[IBIS VER]   4.1
[File Name]   f29h85xpzs.ibs
[File Rev]   1.0
[Date]   May 06, 2024
[Source]   File originated at Texas Instruments
[Copyright]   (c) 2012, Texas Instruments Inc.
[Component]   f29h85xpzs
[Manufacturer]  Texas Instruments
[Package]
| Variable   Typ   Min   Max
R_pkg   2.16E-01   8.19E-02   3.21E-01
L_pkg   3.14E-09   1.61E-09   4.25E-09
C_pkg   1.08E-13   5.34E-14   3.30E-13
[Pin]   signal_name   model_name   R_pin   L_pin   C_pin
1   GPIO15   BQ33100HYPBFZ_PMB_5FS_LC_7LM   2.36E-01   3.63E-09   3.17E-13
2   GPIO16   BCF33100DSHYPBFZ_USF_7LM   2.32E-01   3.55E-09   1.55E-13
3   VDDIO   NC   2.22E-01   3.44E-09   1.06E-13
4   GPIO17   BCF33100DSHYPBFZ_USF_7LM   2.19E-01   3.37E-09   1.03E-13
5   VDD   NC   1.26E-01   2.56E-09   1.03E-13
6   VDD   NC   1.44E-01   2.67E-09   1.01E-13
7   VDDIO   NC   2.99E-01   3.91E-09   9.60E-14
8   GPIO18   BQ33100HYPBFZ_PMB_5FS_LC_7LM   2.79E-01   3.70E-09   9.32E-14
9   GPIO22   BQ33100HYPBFZ_PMB_5FS_LC_7LM   2.67E-01   3.56E-09   9.05E-14
10   B9,GPIO233   BCF33100DSHYPBFZ_USF_7LM   2.79E-01   3.62E-09   8.80E-14
11   B8,GPIO232   BCF33100DSHYPBFZ_USF_7LM   2.61E-01   3.43E-09   8.53E-14
12   A7/E25,GPIO225   BCF33100DSHYPBFZ_USF_7LM   2.73E-01   3.50E-09   8.28E-14
13   A6/E24,GPIO224   BCF33100DSHYPBFZ_USF_7LM   2.58E-01   3.33E-09   8.01E-14
14   VDDA   NC   1.50E-01   2.48E-09   8.54E-14
15   VSSA   NC   1.42E-01   2.46E-09   8.78E-14
16   B3/D27   ICF33SHYPB_LC_7LM   2.76E-01   3.60E-09   8.80E-14
17   B2/D26   ICF33SHYPB_LC_7LM   2.57E-01   3.48E-09   9.04E-14
18   VREFLOAB   NC   1.30E-01   2.47E-09   9.51E-14
19   VREFHIAB   NC   8.60E-02   2.15E-09   9.95E-14
20   A15/B15/C15/D15/E15   ICF33SHYPB_LC_7LM   2.27E-01   3.35E-09   9.80E-14
21   A14/B14/C14/D14/E14   ICF33SHYPB_LC_7LM   2.18E-01   3.32E-09   1.00E-13
22   B1/C27   ICF33SHYPB_LC_7LM   2.14E-01   3.33E-09   1.03E-13
23   B0/C26/VDAC   ICF33SHYPB_LC_7LM   2.16E-01   3.38E-09   1.06E-13
24   A1/C25   ICF33SHYPB_LC_7LM   2.24E-01   3.49E-09   1.55E-13
25   A0/C24/DACA_OUT   ICF33SHYPB_LC_7LM   2.38E-01   3.65E-09   3.17E-13
26   C0/E28   ICF33SHYPB_LC_7LM   2.38E-01   3.71E-09   3.30E-13
27   C1/E29   ICF33SHYPB_LC_7LM   2.23E-01   3.55E-09   1.61E-13
28   D0/B24   ICF33SHYPB_LC_7LM   2.13E-01   3.43E-09   1.57E-13
29   D1/B25   ICF33SHYPB_LC_7LM   2.11E-01   3.37E-09   1.07E-13
30   E0/A24/DACC_OUT   ICF33SHYPB_LC_7LM   2.15E-01   3.36E-09   1.05E-13
31   E1/A25   ICF33SHYPB_LC_7LM   2.23E-01   3.39E-09   1.02E-13
32   VREFLOCDE   NC   1.20E-01   2.50E-09   1.01E-13
33   VREFHICDE   NC   8.67E-02   2.18E-09   1.01E-13
34   D2/B26   ICF33SHYPB_LC_7LM   2.45E-01   3.44E-09   9.40E-14
35   D3/B27   ICF33SHYPB_LC_7LM   2.63E-01   3.55E-09   9.15E-14
36   VSSA   NC   1.41E-01   2.50E-09   9.12E-14
37   VDDA   NC   1.48E-01   2.51E-09   8.87E-14
38   E4/A28,GPIO246   BCF33100DSHYPBFZ_USF_7LM   2.15E-01   3.02E-09   8.30E-14
39   E5/A29,GPIO247   BCF33100DSHYPBFZ_USF_7LM   2.13E-01   2.97E-09   8.02E-14
40   C8,GPIO238   BCF33100DSHYPBFZ_USF_7LM   2.15E-01   2.94E-09   7.76E-14
41   C9,GPIO239   BCF33100DSHYPBFZ_USF_7LM   2.21E-01   2.95E-09   7.49E-14
42   GPIO222/TDI   BCF33100DSHYPBFZ_USF_7LM   2.14E-01   2.85E-09   7.21E-14
43   GPIO223/TDO   BCPF335585DSHYPBFZ_USF_7LM   2.21E-01   2.87E-09   6.95E-14
44   VDDIO   NC   2.31E-01   2.91E-09   6.69E-14
45   VDD   NC   8.84E-02   1.69E-09   6.87E-14
46   VDD3VFL   NC   8.72E-02   1.64E-09   6.59E-14
47   TMS   BCF3355DSHYPBFZ_TMS_USF_7LM   2.47E-01   2.91E-09   5.89E-14
48   TCK   IQ0442FS_40P60P_3X2_USF_7LM   2.66E-01   3.03E-09   5.64E-14
49   VDD   NC   9.94E-02   1.61E-09   5.88E-14
50   GPIO41   BCF33100DSHYPBFZ_CORNER_USF_7LM   2.35E-01   2.69E-09   1.01E-13
51   GPIO219/ERRORSTS   BCF33100DSHYPBFZ_CORNER_USF_7LM   2.61E-01   3.84E-09   3.17E-13
52   VDD3VFL   NC   1.16E-01   2.61E-09   1.61E-13
53   GPIO58   BCF33100DSHYPBFZ_USF_7LM   3.21E-01   4.25E-09   1.07E-13
54   GPIO59   BCF3385DSHYPBFZ_USF_7LM   2.98E-01   4.02E-09   1.04E-13
55   VDD   NC   1.04E-01   2.39E-09   1.06E-13
56   GPIO60   BCF33100DSHYPBFZ_USF_7LM   2.72E-01   3.72E-09   9.83E-14
57   GPIO61   BCF33100DSHYPBFZ_USF_7LM   2.85E-01   3.79E-09   9.59E-14
58   GPIO62   BCF33100DSHYPBFZ_USF_7LM   2.67E-01   3.60E-09   9.31E-14
59   GPIO63   BCF33100DSHYPBFZ_USF_7LM   2.50E-01   3.43E-09   9.04E-14
60   GPIO64   BCF3385DSHYPBFZ_USF_7LM   2.37E-01   3.28E-09   8.77E-14
61   GPIO65   BCF33100DSHYPBFZ_USF_7LM   2.26E-01   3.15E-09   8.50E-14
62   GPIO66   BCF33100DSHYPBFZ_USF_7LM   2.22E-01   3.07E-09   8.24E-14
63   VDDIO   NC   2.20E-01   3.01E-09   7.97E-14
64   GPIO127   BCF33100DSHYPBFZ_USF_7LM   2.25E-01   3.10E-09   8.24E-14
65   VREGENZ   IQ0440FS_VREGENZ_PU_7LM   2.22E-01   3.11E-09   8.49E-14
66   VDD   NC   8.19E-02   2.00E-09   9.14E-14
67   VDDOSC   NC   2.19E-01   3.17E-09   9.01E-14
68   GPIO221,X2   BCPF335585DSHYPBFZ_USF_7LM   2.18E-01   3.20E-09   9.27E-14
69   VSSOSC   NC   2.18E-01   3.24E-09   9.53E-14
70   GPIO220,X1   BCPF335585DSHYPBFZ_USF_7LM   2.22E-01   3.31E-09   9.79E-14
71   XRSn   BQ0491FS_3X2_USF_7LM   2.21E-01   3.34E-09   1.00E-13
72   GPIO38   BCF33100DSHYPBFZ_USF_7LM   2.27E-01   3.44E-09   1.03E-13
73   VDDIO   NC   2.31E-01   3.51E-09   1.06E-13
74   GPIO42   BCPF335585DSHYPBFZ_USF_7LM   2.32E-01   3.56E-09   1.55E-13
75   GPIO43   BCF33100DSHYPBFZ_CORNER_USF_7LM   2.45E-01   3.71E-09   3.17E-13
76   GPIO70   BCF3385DSHYPBFZ_CORNER_7LM   2.49E-01   3.81E-09   3.30E-13
77   GPIO71   BCF33100DSHYPBFZ_USF_7LM   2.34E-01   3.64E-09   1.61E-13
78   VDD   NC   1.22E-01   2.68E-09   1.59E-13
79   VDDIO   NC   2.26E-01   3.49E-09   1.07E-13
80   GPIO72   BCF33100DSHYPBFZ_USF_7LM   2.19E-01   3.39E-09   1.05E-13
81   GPIO84   BCF33100DSHYPBFZ_USF_7LM   2.56E-01   3.66E-09   1.02E-13
82   GPIO31   BCF33100DSHYPBFZ_USF_7LM   2.54E-01   3.60E-09   9.95E-14
83   GPIO30   BCF3355DSHYPBFZ_USF_7LM   2.49E-01   3.51E-09   9.68E-14
84   GPIO29   BQ33100HYPBFZ_PMB_5FS_LC_7LM   2.43E-01   3.43E-09   9.40E-14
85   GPIO26   BCF33100DSHYPBFZ_USF_7LM   2.72E-01   3.62E-09   9.16E-14
86   GPIO25   BCF33100DSHYPBFZ_USF_7LM   2.54E-01   3.43E-09   8.87E-14
87   GPIO23   BQ33100HYPBFZ_PMB_5FS_LC_7LM   2.45E-01   3.31E-09   8.59E-14
88   GPIO0   BCF33100DSHYPBFZ_USF_7LM   2.47E-01   3.29E-09   8.32E-14
89   GPIO1   BCF33100DSHYPBFZ_USF_7LM   2.34E-01   3.14E-09   8.04E-14
90   GPIO2   BCF33100DSHYPBFZ_USF_7LM   2.23E-01   3.01E-09   7.76E-14
91   GPIO3   BCF33100DSHYPBFZ_USF_7LM   2.16E-01   2.91E-09   7.49E-14
92   GPIO4   BCF33100DSHYPBFZ_USF_7LM   2.13E-01   2.84E-09   7.21E-14
93   GPIO5   BCF33100DSHYPBFZ_USF_7LM   2.12E-01   2.79E-09   6.94E-14
94   GPIO6   BCF3355DSHYPBFZ_USF_7LM   2.16E-01   2.78E-09   6.68E-14
95   VDD   NC   1.19E-01   1.94E-09   6.61E-14
96   GPIO8   BCF33100DSHYPBFZ_USF_7LM   2.15E-01   2.69E-09   6.13E-14
97   GPIO9   BCF3385DSHYPBFZ_USF_7LM   2.22E-01   2.71E-09   5.87E-14
98   GPIO10   BQ33100HYPBFZ_PMB_5FS_LC_7LM   2.26E-01   2.70E-09   5.60E-14
99   GPIO11   BCF33100DSHYPBFZ_USF_7LM   2.36E-01   2.74E-09   5.34E-14
100   GPIO12   BCF33100DSHYPBFZ_CORNER_USF_7LM   2.47E-01   2.79E-09   1.02E-13
| End of package information
|   Component BCF33100DSHYPBFZ_7LM
[Component]   BCF33100DSHYPBFZ_7LM
[Manufacturer]  IO Methodology Inc.
[Package]
|   typ   min   max
R_pkg   0   0   0
L_pkg   0   0   0
C_pkg   0   0   0
[Pin]   signal_name  model_name   R_pin   L_pin   C_pin
VSS   VSS   GND
VDDS   VDDS   POWER
PAD   PAD   BCF33100DSHYPBFZ_7LM
[Model Selector] BCF33100DSHYPBFZ_7LM
WK_PU_ON_3P3  Cell operated at 3.3(nom)
|WK_PU_ON_3P3; WEAK_PULLUP_ON
WK_PD_ON_3P3  Cell operated at 3.3(nom)
|WK_PD_ON_3P3; WEAK_PULLDOWN_ON
DRIVER_MODE_3P3  Cell operated at 3.3(nom)
|DRIVER_MODE_3P3
RECEIVER_MODE_3P3  Cell operated at 3.3(nom)
|   Component BCF33100DSHYPBFZ_USF_7LM
[Component]   BCF33100DSHYPBFZ_USF_7LM
[Manufacturer]  Texas Instruments
[Package]
| variable   typ   min   max
R_pkg   0.0   0.0   0.0
L_pkg   0.0H   0.0H   0.0H
C_pkg   0.0F   0.0F   0.0F
[Pin]  signal_name   model_name   R_pin   L_pin   C_pin
PAD   PAD   BCF33100_USF_7LM_IO_3.3V   0   0   0
VDDS   VDDS   Power   0   0   0
VSS   VSS   Gnd   0   0   0
[Model Selector] BCF33100DSHYPBFZ_USF_7LM
BCF33100_USF_7LM_IO_3.3V I/O model with 3.3V supply
|   Component BCF33100DSHYPBFZ_CORNER_USF_7LM
[Component]   BCF33100DSHYPBFZ_CORNER_USF_7LM
[Manufacturer]  Texas Instruments
[Package]
| variable   typ   min   max
R_pkg   0.0   0.0   0.0
L_pkg   0.0H   0.0H   0.0H
C_pkg   0.0F   0.0F   0.0F
[Pin]  signal_name   model_name   R_pin   L_pin   C_pin
PAD   PAD   BCF33100_CORNER_7LM_IO_3.3V   0   0   0
VDDS   VDDS   Power   0   0   0
VSS   VSS   Gnd   0   0   0
[Model Selector] BCF33100DSHYPBFZ_CORNER_USF_7LM
BCF33100_CORNER_7LM_IO_3.3V  I/O model with 3.3V supply
|   Component BCF3355DSHYPBFZ_TMS_USF_7LM
[Component]   BCF3355DSHYPBFZ_TMS_USF_7LM
[Manufacturer]  Texas Instruments
[Package]
| variable   typ   min   max
R_pkg   0.0   0.0   0.0
L_pkg   0.0H   0.0H   0.0H
C_pkg   0.0F   0.0F   0.0F
[Pin]  signal_name   model_name   R_pin   L_pin   C_pin
PAD   PAD   BCF3355_TMS_7LM_IO_3.3V   0   0   0
VDDS   VDDS   Power   0   0   0
VSS   VSS   Gnd   0   0   0
[Model Selector] BCF3355DSHYPBFZ_TMS_USF_7LM
BCF3355_TMS_7LM_IO_3.3V I/O model with 3.3V supply
|   Component IQ0442FS_40P60P_3X2_USF_7LM
[Component]   IQ0442FS_40P60P_3X2_USF_7LM
[Manufacturer]  Texas Instruments
[Package]
| variable   typ   min   max
R_pkg   0.0   0.0   0.0
L_pkg   0.0H   0.0H   0.0H
C_pkg   0.0F   0.0F   0.0F
[Pin]  signal_name   model_name   R_pin   L_pin   C_pin
PAD   PAD   IQRX_3.3V   0   0   0
VDDS   VDDS   Power   0   0   0
VSS   VSS   Gnd   0   0   0
[Model Selector] IQ0442FS_40P60P_3X2_USF_7LM
IQRX_3.3V I/O model with 3.3V supply
|   Component BCF3355DSHYPBFZ_USF_7LM
[Component]   BCF3355DSHYPBFZ_USF_7LM
[Manufacturer]  Texas Instruments
[Package]
| variable   typ   min   max
R_pkg   0.0   0.0   0.0
L_pkg   0.0H   0.0H   0.0H
C_pkg   0.0F   0.0F   0.0F
[Pin]  signal_name   model_name   R_pin   L_pin   C_pin
PAD   PAD   BCF3355_USF_7LM_IO_3.3V   0   0   0
VDDS   VDDS   Power   0   0   0
VSS   VSS   Gnd   0   0   0
[Model Selector] BCF3355DSHYPBFZ_USF_7LM
BCF3355_USF_7LM_IO_3.3V I/O model with 3.3V supply
|   Component BCF3385DSHYPBFZ_CORNER_7LM
[Component]   BCF3385DSHYPBFZ_CORNER_7LM
[Manufacturer]  IO Methodology Inc.
[Package]
|   typ   min   max
R_pkg   0   0   0
L_pkg   0   0   0
C_pkg   0   0   0
[Pin]   signal_name  model_name   R_pin   L_pin   C_pin
VSS   VSS   GND
VDDS   VDDS   POWER
PAD   PAD   BCF3385DSHYPBFZ_CORNER_7LM
[Model Selector] BCF3385DSHYPBFZ_CORNER_7LM
WK_PU_ON_3P3_BCF3385DSHYPBFZ_CORNER_7LM  Cell operated at 3.3(nom)
|WK_PU_ON_3P3; WEAK_PULLUP_ON
WK_PD_ON_3P3_BCF3385DSHYPBFZ_CORNER_7LM  Cell operated at 3.3(nom)
|WK_PD_ON_3P3; WEAK_PULLDOWN_ON
DRIVER_MODE_3P3_BCF3385_CORNER_7LM Cell operated at 3.3(nom)
|DRIVER_MODE_3P3
RECEIVER_MODE_3P3_BCF3385_CORNER_7LM  Cell operated at 3.3(nom)
|   Component BCF3385DSHYPBFZ_USF_7LM
[Component]   BCF3385DSHYPBFZ_USF_7LM
[Manufacturer]  Texas Instruments
[Package]
| variable   typ   min   max
R_pkg   0.0   0.0   0.0
L_pkg   0.0H   0.0H   0.0H
C_pkg   0.0F   0.0F   0.0F
[Pin]  signal_name   model_name   R_pin   L_pin   C_pin
PAD   PAD   BCF3385_USF_7LM_IO_3.3V   0   0   0
VDDS   VDDS   Power   0   0   0
VSS   VSS   Gnd   0   0   0
[Model Selector] BCF3385DSHYPBFZ_USF_7LM
BCF3385_USF_7LM_IO_3.3V I/O model with 3.3V supply
|   Component BCPF335585DSHYPBFZ_USF_7LM
[Component]   BCPF335585DSHYPBFZ_USF_7LM
[Manufacturer]  Texas Instruments
[Package]
| variable   typ   min   max
R_pkg   0.0   0.0   0.0
L_pkg   0.0H   0.0H   0.0H
C_pkg   0.0F   0.0F   0.0F
[Pin]  signal_name   model_name   R_pin   L_pin   C_pin
PAD   PAD   BCPF335585DSHYPBFZ_USF_7LM   0   0   0
VDDS   VDDS   Power   0   0   0
VSS   VSS   Gnd   0   0   0
[Model Selector]   BCPF335585DSHYPBFZ_USF_7LM
BCPF335585_7LM_IO_DS0_3.3V   I/O model DS 0 with 3.3V supply
BCPF335585_7LM_IO_DS1_3.3V   I/O model DS 1 with 3.3V supply
|   Component BQ0491FS_3X2_USF_7LM
[Component]   BQ0491FS_3X2_USF_7LM
[Manufacturer]  Texas Instruments
[Package]
| variable   typ   min   max
R_pkg   0.0   0.0   0.0
L_pkg   0.0H   0.0H   0.0H
C_pkg   0.0F   0.0F   0.0F
[Pin]  signal_name   model_name   R_pin   L_pin   C_pin
PAD   PAD   BQ0491FS_3X2_USF_7LM   0   0   0
VDDS   VDDS   Power   0   0   0
VSS   VSS   Gnd   0   0   0
[Model Selector]   BQ0491FS_3X2_USF_7LM
BQ0491_3X2_USF_7LM_IO_15p_3p3   I/O open drain model with C_fixture 15pF for 3.3V supply
BQ0491_3X2_USF_7LM_IO_50p_3p3   I/O open drain model with C_fixture 50pF for 3.3V supply
BQ0491_3X2_USF_7LM_IO_100p_3p3   I/O open drain model with C_fixture 100pF for 3.3V supply
BQ0491_3X2_USF_7LM_IO_150p_3p3   I/O open drain model with C_fixture 150pF for 3.3V supply
|   Component BQ33100HYPBFZ_PMB_5FS_LC_7LM
[Component]   BQ33100HYPBFZ_PMB_5FS_LC
[Manufacturer]  Texas Instruments
[Package]
| variable   typ   min   max
R_pkg   0.0   0.0   0.0
L_pkg   0.0H   0.0H   0.0H
C_pkg   0.0F   0.0F   0.0F
[Pin]  signal_name   model_name   R_pin   L_pin   C_pin
Pin1   PAD   BQ33100HYPBFZ_PMB_5FS_LC_7LM   0   0   0
Pin2   VDDS   Power   0   0   0
Pin3   VSS   Gnd   0   0   0
[Model Selector]   BQ33100HYPBFZ_PMB_5FS_LC_7LM
BQ33_PMB_IO_M0_D0   I/O model with Mode = 0 and Drive = 0
BQ33_PMB_IO_M0_D1   I/O model with Mode = 0 and Drive = 1
BQ33_PMB_IO_M1_D0   I/O model with Mode = 1 and Drive = 0
BQ33_PMB_IO_M1_D1   I/O model with Mode = 1 and Drive = 1
|   Component IQ0440FS_VREGENZ_PU_7LM
[Component]   IQ0440FS_VREGENZ_PU_7LM
[Manufacturer]  Texas Instruments
[Package]
|   typ   min   max
R_pkg   0   0   0
L_pkg   0   0   0
C_pkg   0   0   0
[Pin]   signal_name  model_name   R_pin   L_pin   C_pin
VSS   VSS   GND
VDDS   VDDS   POWER
PAD   PAD   IQ0440FS_VREGENZ_PU_7LM
[Model Selector] IQ0440FS_VREGENZ_PU_7LM
WK_PD_ON_3P3_IQ0440FS_VREGENZ_PU_7LM Cell operated at 3.3(nom)
|WK_PD_ON_3P3; WEAK_PULLDOWN_ON
RECEIVER_MODE_3P3_IQ0440FS_VREGENZ  Cell operated at 3.3(nom)
|   Component ICF33SHYPB_LC_7LM
[Component]   ICF33SHYPB_LC_7LM
[Manufacturer]   Texas Instruments
[Package]
|  variable   typ   min   max
R_pkg   0   0   0
L_pkg   0   0   0
C_pkg   0   0   0
[Pin]   signal_name   model_name   R_pin   L_pin   C_pin
VSS   VSS   GND
VDDS   VDDS   POWER
PAD   PAD   ICF33SHYPB_LC_7LM
[Model Selector] ICF33SHYPB_LC_7LM
RECEIVER_MODE_3P3_ICF_7LM  Cell operated at 3.3(nom)
|RECEIVER_MODE_3P3_ICF_7LM; RECEIVER_MODE
WK_PU_ON_3P3_ICF_7LM  Cell operated at 3.3(nom)
|WK_PU_ON_3P3_ICF_7LM; WEAK_PULLUP_ON
WK_PD_ON_3P3_ICF_7LM  Cell operated at 3.3(nom)
| Models and submodels in the file (29): WK_PU_ON_3P3 (Input), WK_PD_ON_3P3 (Input), DRIVER_MODE_3P3 (I/O), RECEIVER_MODE_3P3 (Input), BCF33100_USF_7LM_IO_3.3V (I/O), BCF33100_CORNER_7LM_IO_3.3V (I/O), BCF3355_TMS_7LM_IO_3.3V (I/O), IQRX_3.3V (Input), BCF3355_USF_7LM_IO_3.3V (I/O), WK_PU_ON_3P3_BCF3385DSHYPBFZ_CORNER_7LM (Input), WK_PD_ON_3P3_BCF3385DSHYPBFZ_CORNER_7LM (Input), DRIVER_MODE_3P3_BCF3385_CORNER_7LM (I/O), RECEIVER_MODE_3P3_BCF3385_CORNER_7LM (Input), BCF3385_USF_7LM_IO_3.3V (I/O), BCPF335585_7LM_IO_DS0_3.3V (I/O), BCPF335585_7LM_IO_DS1_3.3V (I/O), BQ0491_3X2_USF_7LM_IO_15p_3p3 (I/O_open_drain), BQ0491_3X2_USF_7LM_IO_50p_3p3 (I/O_open_drain), BQ0491_3X2_USF_7LM_IO_100p_3p3 (I/O_open_drain), BQ0491_3X2_USF_7LM_IO_150p_3p3 (I/O_open_drain), BQ33_PMB_IO_M0_D0 (I/O), BQ33_PMB_IO_M0_D1 (I/O), BQ33_PMB_IO_M1_D0 (I/O), BQ33_PMB_IO_M1_D1 (I/O), WK_PD_ON_3P3_IQ0440FS_VREGENZ_PU_7LM (Input), RECEIVER_MODE_3P3_IQ0440FS_VREGENZ (Input), RECEIVER_MODE_3P3_ICF_7LM (Input), WK_PU_ON_3P3_ICF_7LM (Input), WK_PD_ON_3P3_ICF_7LM (Input)
